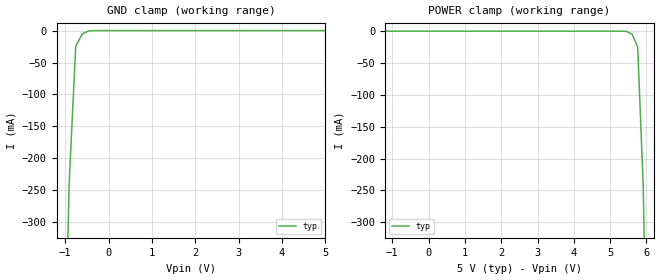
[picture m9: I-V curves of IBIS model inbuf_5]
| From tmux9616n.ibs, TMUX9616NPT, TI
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| inbuf_5
[Model]   inbuf_5
Model_type   Input
Vinl = 1.5
Vinh = 3
|   typ   min   max
C_comp   1.598234e-12   NA   NA
[Voltage Range]   5   NA   NA
[Temperature Range]   27   NA   NA
[Power Clamp Reference]   5   NA   NA
[GND Clamp Reference]   0   NA   NA
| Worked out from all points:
|   GND clamp passes 1 mA (typ) near -0.47 V on its own axis
[GND Clamp]
|   Voltage   I(typ)   I(min)   I(max)
-10V      -41.03A    NA         NA
-1.061V   -698.9mA   NA         NA
-909.1mV  -240.8mA   NA         NA
-757.6mV  -24.8mA    NA         NA
-606.1mV  -5.055mA   NA         NA
-454.5mV  -460.8uA   NA         NA
-303mV    -5.768uA   NA         NA
5V        526.9nA    NA         NA
[POWER Clamp]
|   Voltage   I(typ)   I(min)   I(max)
-5V       947.4uA    NA         NA
5.455V    -460.8uA   NA         NA
5.606V    -5.055mA   NA         NA
5.758V    -24.8mA    NA         NA
5.909V    -240.8mA   NA         NA
6.061V    -698.9mA   NA         NA
10V       -17.96A    NA         NA
